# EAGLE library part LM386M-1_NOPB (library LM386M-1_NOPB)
Wide Input Voltage Low Power Audio Amplifier with Internal Gain Source: Datasheet
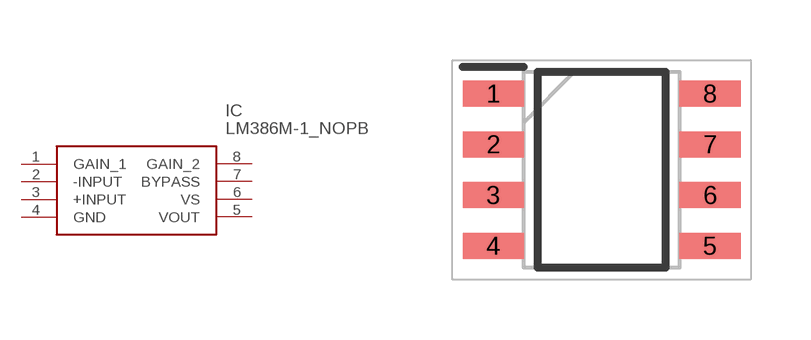
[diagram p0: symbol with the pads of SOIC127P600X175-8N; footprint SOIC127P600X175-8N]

Designator prefix IC

## LM386M-1_NOPB (Arrow_Part_Number: LM386M-1/NOPB; Arrow_Price-Stock: https://www.arrow.com/en/products/lm386m-1nopb/texas-instruments?region=nac; Description: Wide Input Voltage Low Power Audio Amplifier with Internal Gain; Height: 1.75mm; Manufacturer_Name: Texas Instruments; Manufacturer_Part_Number: LM386M-1/NOPB; Mouser_Part_Number: 926-LM386M-1/NOPB; Mouser_Price-Stock: https://www.mouser.co.uk/ProductDetail/Texas-Instruments/LM386M-1-NOPB?qs=QbsRYf82W3GaJvrwUmrW3g%3D%3D)  [SOIC127P600X175-8N]
1  GAIN_1
2  -INPUT
3  +INPUT
4  GND
5  VOUT
6  VS
7  BYPASS
8  GAIN_2

## Footprint SOIC127P600X175-8N (pad centres in mm)
+soic d
smd 1.528 x 0.65: 1 -2.711,1.905; 2 -2.711,0.635; 3 -2.711,-0.635; 4 -2.711,-1.905; 5 2.711,-1.905; 6 2.711,-0.635; 7 2.711,0.635; 8 2.711,1.905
